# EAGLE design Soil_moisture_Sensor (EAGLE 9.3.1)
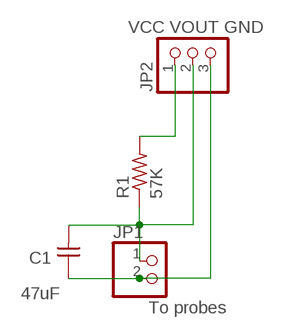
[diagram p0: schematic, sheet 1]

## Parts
C1  47uF  CAP-UNPOLARIZED  [C1206]
JP1  To probes  PINHD-1X02_2.54-SMD  [1X02SMD]
JP2  VCC VOUT GND  PINHD-1X03_2.54-SMD  [1X03SMD]
R1  57K  RES-US1206  [R1206]

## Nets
N$1: JP2.1 R1.2
N$2: C1.1 JP1.2 JP2.3
N$4: C1.2 JP1.1 JP2.2 R1.1

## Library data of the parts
C1 = eagle_fab:CAP-UNPOLARIZED
JP1 = pinhead-2:PINHD-1X02: PIN HEADER
JP2 = pinhead-2:PINHD-1X03: PIN HEADER
R1 = eagle_fab:RES-US: Resistor (US Symbol)

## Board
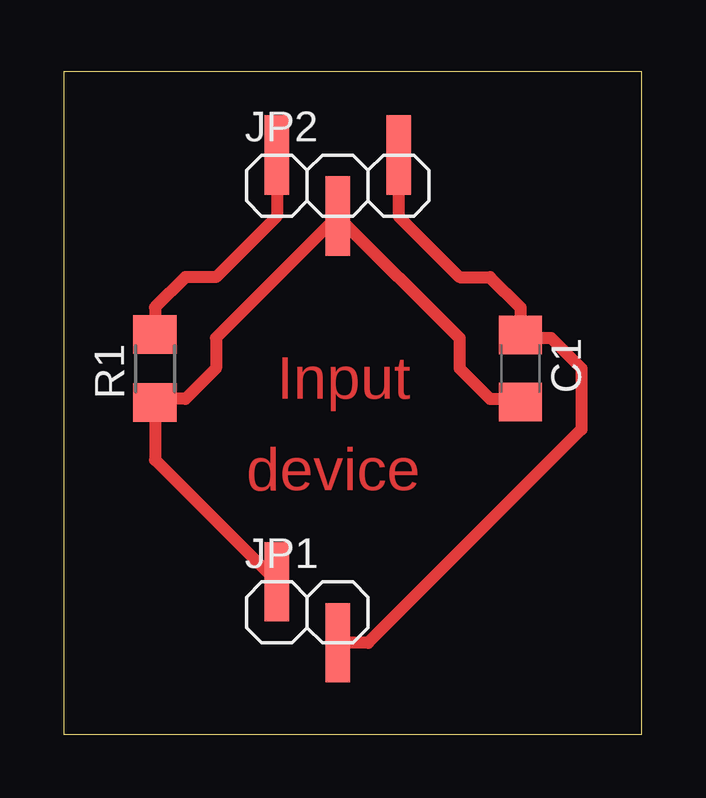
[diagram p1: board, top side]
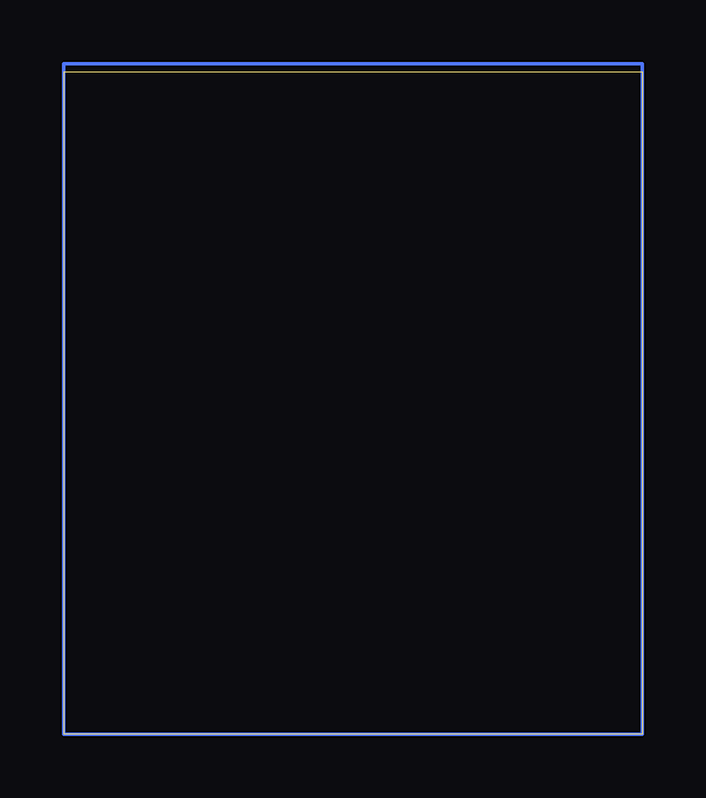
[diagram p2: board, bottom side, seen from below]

Size 24.11 x 27.61 mm. Coordinates in mm from the lower left corner, seen from the top.
Outline: 0,0 24.11,0 24.11,27.61 0,27.61 0,0
Copper layers (1*16): Top 0.035mm / dielectric 1.5mm / Bottom 0.035mm
Design rules "default": minimum track width 6mil, minimum drill 0.35mm, track to track 6mil, track to pad 6mil, pad to pad 6mil, via to via 6mil, smd to smd 6mil, copper to edge 40mil, drill to drill 6mil, minimum pad ring 10mil, minimum via ring 8mil, stop-mask expansion 4mil, vias tented up to drill 0mil, thermal gap 10mil

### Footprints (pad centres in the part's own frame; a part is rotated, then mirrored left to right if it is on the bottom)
C1206 = smd 1.6 x 1.8: 1 -1.4,0; 2 1.4,0
1X02SMD = smd 1.016 x 3.302: 1 -1.27,1.27; 2 1.27,-1.27
1X03SMD = smd 1.016 x 3.302: 1 -1.27,1.27; 2 1.27,-1.27; 3 3.81,1.27
R1206 = smd 1.6 x 1.803: 1 -1.422,0; 2 1.422,0

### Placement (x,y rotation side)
C1  19.05,15.24 270 top
JP1  10.16,5.08 0 top
JP2  10.16,22.86 0 top
R1  3.81,15.24 90 top

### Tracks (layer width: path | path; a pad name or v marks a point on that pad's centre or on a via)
N$1
  Top 0.508: JP2.1 8.89,21.59 6.35,19.05 5.08,19.05 3.81,17.78 R1.2
N$2
  Top 0.508: JP2.3 13.97,21.59 16.51,19.05 17.78,19.05 19.05,17.78 C1.1 19.18,16.51 20.32,16.51 21.59,15.24 21.59,12.7 12.7,3.81 JP1.2
N$3
  Bottom 0.152: 0,27.94 24.13,27.94 24.13,0 0,0 0,27.94
N$4
  Top 0.152: 8.89,7.62 JP1.1 | 19.06,13.97 C1.2 | R1.1 3.96,13.97
  Top 0.508: 19.06,13.97 17.78,13.97 16.51,15.24 16.51,16.51 JP2.2 6.35,16.51 6.35,15.24 5.08,13.97 3.96,13.97 R1.1 3.81,11.43 JP1.1

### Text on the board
Top: Input | device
